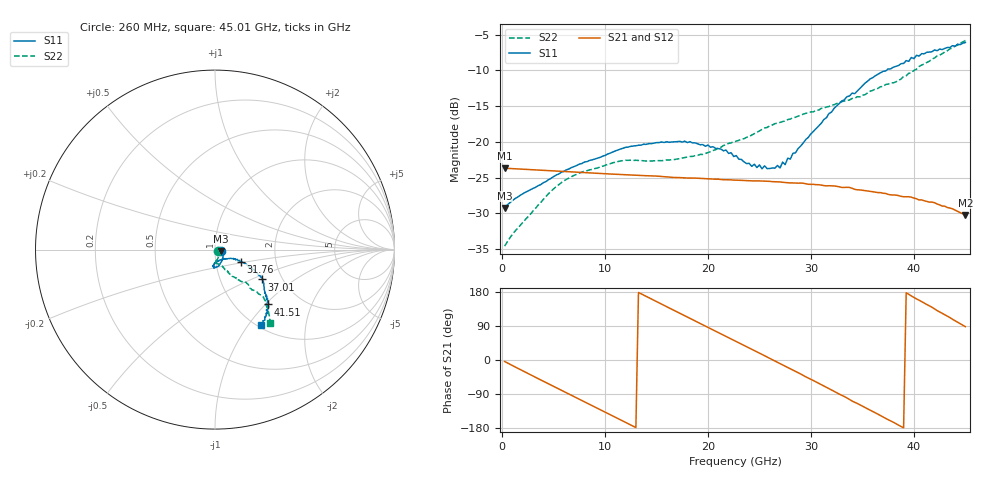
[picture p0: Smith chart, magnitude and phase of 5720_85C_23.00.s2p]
! Device:  ADRF5720
! Description: 0.5dB LSB GaAs MMIC 6-bit Digital Attenuator
! Frequency:  0.000009 -  40 GHz
! Ports:
!	RF1	= Port 1
!	RF2	= Port 2
! Vdd:  3.3 Volt
! Vss:  -3.3 Volt
! Control:  0/3.3 Volt
! State:  23.00 dB attenuation
! Data:  The device was measured using G-S-G Probes on a matrix board.
!  Data was collected using an calibrated 4 port network analyzer.
!  The reference plane for this measurement is at the launchers.
! Note:  Analog Devices supplies this data as a sample of measured data
!  for this product.  Your particular data for this product may vary.
!  Data was taken at 85 degrees C.
!  Analog Devices reserves the right to change this data at anytime.
# GHZ S DB R 45.0
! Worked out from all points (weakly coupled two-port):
!   180 points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, 260 MHz to 45.01 GHz, reference 45 ohm
!   highest |S21| = -23.69 dB at 260 MHz (marker M1); lowest = -30.2 dB at 45.01 GHz (marker M2)
!   lowest |S11| = -29.3 dB at 260 MHz (marker M3), VSWR 1.07, Z = 48.1 - j0.787 ohm
!   |S11| at or under -10 dB: start of sweep to 37.35 GHz
!   |S22| runs from -34.6 to -5.8 dB; largest |S21 - S12| = 0.00039
!   S11 on the Smith chart (normalised r, x): 260 MHz: 1.07, -0.02; 31.76 GHz: 1.32, -0.18; 37.01 GHz: 1.58, -0.58; 41.51 GHz: 1.38, -1.03; 45.01 GHz: 1.03, -1.16
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0.26  -29.26 -13.7  -23.69 -3.8  -23.68 -3.8  -34.59 -26.0
1.26  -27.95 -3.9  -23.77 -18.0  -23.76 -18.0  -32.50 -13.7
4.76  -25.11 -36.6  -24.04 -66.2  -24.02 -66.1  -26.92 -65.2
7.76  -23.04 -55.0  -24.28 -107.0  -24.26 -106.9  -24.25 -81.5
11.51  -21.01 -74.1  -24.57 -157.9  -24.56 -157.8  -22.67 -92.5
15.26  -20.11 -87.1  -24.82 150.7  -24.81 150.8  -22.63 -90.8
18.26  -19.98 -94.2  -25.06 110.1  -25.05 110.3  -22.05 -82.3
22.76  -21.93 -91.7  -25.36 48.7  -25.34 48.9  -19.91 -67.3
24.26  -23.43 -84.8  -25.46 28.4  -25.45 28.6  -19.05 -64.3
27.01  -23.65 -53.5  -25.61 -9.6  -25.59 -9.3  -17.29 -60.0
27.26  -22.84 -48.4  -25.66 -13.1  -25.64 -12.9  -17.17 -60.5
27.51  -23.19 -47.0  -25.69 -16.4  -25.68 -16.1  -17.09 -59.5
27.76  -22.28 -42.3  -25.71 -19.8  -25.70 -19.5  -16.89 -60.2
28.01  -22.42 -42.3  -25.75 -23.3  -25.74 -23.0  -16.82 -59.6
30.26  -18.53 -27.4  -25.95 -54.4  -25.93 -54.1  -15.81 -58.5
31.76  -16.05 -25.2  -26.14 -75.1  -26.12 -74.8  -15.06 -57.1
34.51  -12.90 -25.9  -26.71 -114.6  -26.68 -114.3  -13.69 -53.1
37.01  -10.15 -32.3  -27.19 -150.3  -27.17 -150.0  -12.28 -47.4
37.76  -9.81 -33.8  -27.42 -161.0  -27.40 -160.6  -11.76 -46.7
41.51  -7.46 -46.2  -28.43 143.0  -28.40 143.4  -8.73 -44.4
43.51  -6.81 -50.5  -29.26 111.9  -29.23 112.3  -6.99 -48.7
45.01  -6.11 -58.7  -30.22 87.9  -30.20 88.3  -5.83 -53.2
